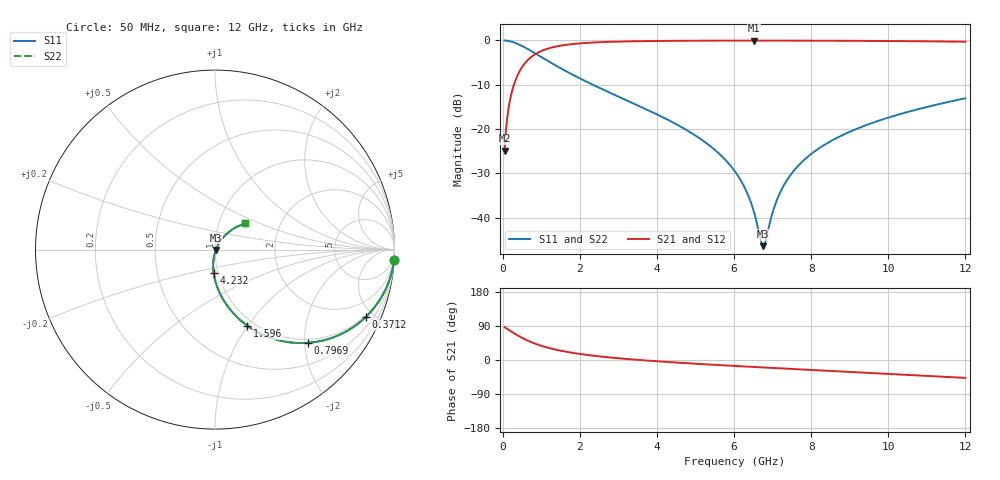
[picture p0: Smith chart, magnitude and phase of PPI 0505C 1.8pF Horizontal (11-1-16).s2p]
# GHz S MA R 50
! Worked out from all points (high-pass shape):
!   1601 points, 50 MHz to 12 GHz, reference 50 ohm
!   highest |S21| = -0.04 dB at 6.51 GHz (marker M1); lowest = -24.9 dB at 50 MHz (marker M2)
!   |S21| within 3 dB of the highest: 856.1 MHz to end of sweep
!   lowest |S11| = -46.4 dB at 6.757 GHz (marker M3), VSWR 1.01, Z = 50.4 - j0.172 ohm
!   |S11| at or under -10 dB: 2.337 GHz to end of sweep
!   |S22| runs from -46.4 to 0.0 dB; largest |S21 - S12| = 0
!   S11 on the Smith chart (normalised r, x): 50 MHz: 1, -33; 371.2 MHz: 0.92, -4.49; 796.9 MHz: 0.92, -2.07; 1.596 GHz: 0.92, -1.00; 4.232 GHz: 0.95, -0.25; 12 GHz: 1.33, +0.41
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0.05  0.9984 -3.4  0.05718 86.6  0.05718 86.6  0.9984 -3.4
0.1919063  0.9766 -13.0  0.2148 77.0  0.2148 77.0  0.9766 -13.0
0.3711563  0.9197 -24.2  0.392 65.8  0.392 65.8  0.9197 -24.2
0.796875  0.7338 -45.0  0.6779 44.9  0.6779 44.9  0.7338 -45.0
1.170313  0.5869 -57.3  0.8077 32.5  0.8077 32.5  0.5869 -57.3
1.596031  0.4608 -67.0  0.8851 22.7  0.8851 22.7  0.4608 -67.0
2.044156  0.3648 -74.2  0.9283 15.4  0.9283 15.4  0.3648 -74.2
4.038312  0.1439 -92.2  0.9857 -3.6  0.9857 -3.6  0.1439 -92.2
4.2325  0.1306 -93.3  0.9874 -4.9  0.9874 -4.9  0.1306 -93.3
5.322938  0.06737 -98.2  0.9932 -11.8  0.9932 -11.8  0.06737 -98.2
6.025  0.03321 -98.0  0.9946 -15.7  0.9946 -15.7  0.03321 -98.0
6.301344  0.02075 -94.5  0.9948 -17.3  0.9948 -17.3  0.02075 -94.5
6.510469  0.01185 -85.2  0.9948 -18.4  0.9948 -18.4  0.01185 -85.2
6.689719  0.00563 -51.8  0.9948 -19.4  0.9948 -19.4  0.00563 -51.8
6.756938  0.004783 -20.8  0.9948 -19.7  0.9948 -19.7  0.004783 -20.8
6.824156  0.005573 10.3  0.9947 -20.1  0.9947 -20.1  0.005573 10.3
7.055688  0.01365 47.6  0.9946 -21.3  0.9946 -21.3  0.01365 47.6
7.264812  0.02215 54.5  0.9943 -22.4  0.9943 -22.4  0.02215 54.5
8.019156  0.05313 57.9  0.9928 -26.4  0.9928 -26.4  0.05313 57.9
8.855656  0.08729 55.6  0.9899 -30.7  0.9899 -30.7  0.08729 55.6
10.01331  0.1352 50.7  0.984 -36.7  0.984 -36.7  0.1352 50.7
12  0.2225 40.9  0.9669 -47.2  0.9669 -47.2  0.2225 40.9
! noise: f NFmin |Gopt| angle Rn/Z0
0.05  0.0008681  0.952  1.755  0.004059
1.372  0.005782  0.7648  5.336  0.004984
2.701  0.009226  0.7168  8.861  0.006402
4.031  0.01228  0.6883  12.45  0.007573
5.36  0.01517  0.6693  16.03  0.008652
6.682  0.01798  0.6565  19.54  0.009705
8.012  0.02081  0.6481  23.01  0.01079
9.341  0.0237  0.6434  26.42  0.01195
10.67  0.02671  0.6419  29.76  0.01321
12  0.02988  0.6431  33.04  0.01462
